(* Logix 5000 Program export KEP; software revision 30.00; part 11 of 15 *)
(* tags used below, declared in another part *)
   EdDSA_INTERNAL : EdDSA_INTERNAL[5];
   EdDSA_STATES : EdDSA_STATECTRL[15];
   InternalFlags : InternalFlags[5];
   InternalFlag_AllNodesUsingKsPrime : BOOL;
   InternalFlag_CreateNewKsPrime : BOOL;
   InternalFlag_KeyServerIdentityNo : BOOL;
   InternalFlag_KeyServerIdentityYes : BOOL;
   InternalFlag_KsEqualKsPrimeStatus : BOOL;
   InternalFlag_KsExists : BOOL;
   InternalFlag_KsIDMatchesServer : BOOL;
   InternalFlag_KsPrimeAvail : BOOL;
   InternalFlag_KsPrimeExists : BOOL;
   InternalFlag_KsPrimeIDMatchesServer : BOOL;
   InternalFlag_PowerOnCycle : BOOL;
   Internal_EdDSA_Msg : EdDSA_MSG;
   KsPrimeExchangeErrorTimer : TIMER;
   MyNodeNumber : DINT;
   ProcessorState : DINT;
   ServerNode : INT;
   T_INT1 : INT;
   WorkingNode : DINT;
   EdDSA_KS : DINT[8];
   EdDSA_KS_Prime : DINT[8];
   EdDSA_MSG_NODE_BLANK : EdDSA_MSG;
   EdDSA_MSG_TO_NODE1 : EdDSA_MSG;
   EdDSA_MSG_TO_NODE2 : EdDSA_MSG;
   EdDSA_MSG_TO_NODE3 : EdDSA_MSG;
   EdDSA_MSG_TO_NODE4 : EdDSA_MSG;
   FirstScan_EdDSA : BOOL;
   InternalFlag_AllNodesHaveMyKs : BOOL;
   InternalFlag_AllNodesHaveMyKsPrime : BOOL;
   InternalFlag_KsID : LINT;
   InternalFlag_KsPrimeID : LINT;
   NODE : VMAC_DATA_INTERNAL[5];
   Wrk_InpA : DINT[2];
   Wrk_InpB : DINT[2];
(* KEP, continued *)

ROUTINE MainRoutine   (* ladder *)
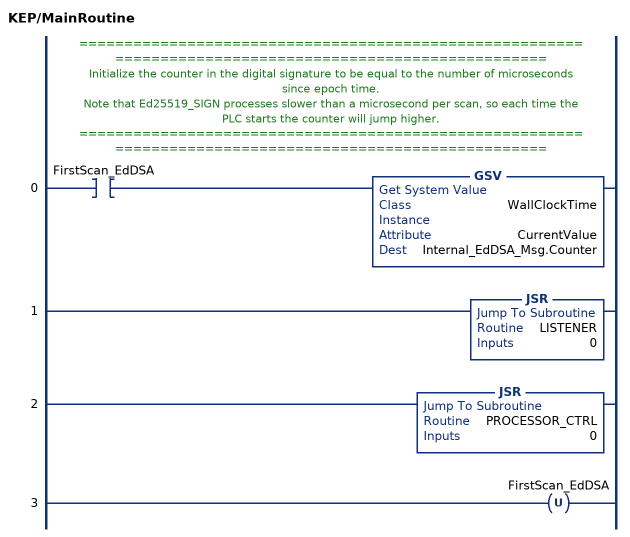
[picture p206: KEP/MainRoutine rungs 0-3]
   // ========================================================================================================
   // Initialize the counter in the digital signature to be equal to the number of microseconds since epoch time.
   // Note that Ed25519_SIGN processes slower than a microsecond per scan, so each time the PLC starts the counter will jump higher.
   // ========================================================================================================
   0: XIC(FirstScan_EdDSA)GSV(WallClockTime,,CurrentValue,Internal_EdDSA_Msg.Counter);
   1: JSR(LISTENER,0);
   2: JSR(PROCESSOR_CTRL,0);
   3: OTU(FirstScan_EdDSA);
END_ROUTINE

ROUTINE PROCESSOR_CTRL   (* ladder *)
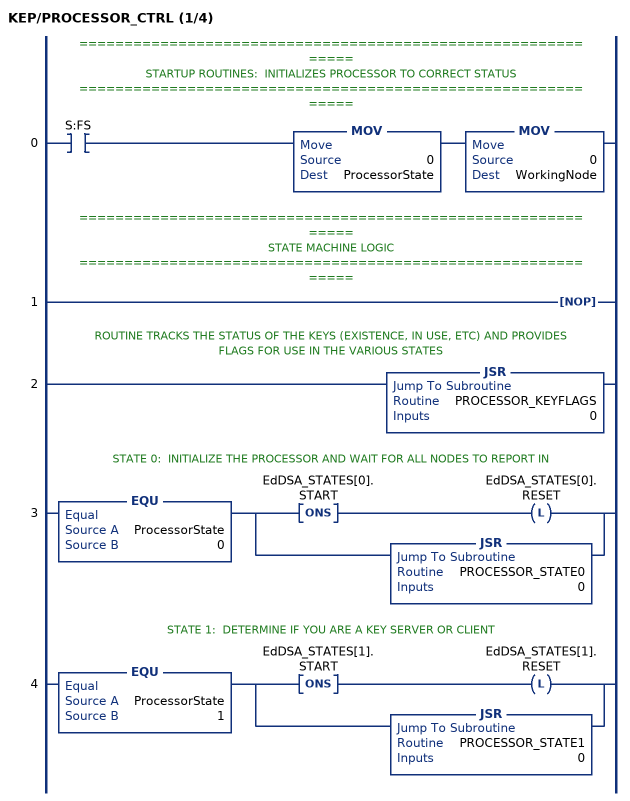
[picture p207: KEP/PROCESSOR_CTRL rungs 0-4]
   // =============================================================
   // STARTUP ROUTINES:  INITIALIZES PROCESSOR TO CORRECT STATUS
   // =============================================================
   0: XIC(S:FS)MOV(0,ProcessorState)MOV(0,WorkingNode);
   // =============================================================
   // STATE MACHINE LOGIC
   // =============================================================
   1: NOP();
   // ROUTINE TRACKS THE STATUS OF THE KEYS (EXISTENCE, IN USE, ETC) AND PROVIDES FLAGS FOR USE IN THE VARIOUS STATES
   2: JSR(PROCESSOR_KEYFLAGS,0);
   // STATE 0:  INITIALIZE THE PROCESSOR AND WAIT FOR ALL NODES TO REPORT IN
   3: EQU(ProcessorState,0)[ONS(EdDSA_STATES[0].START) OTL(EdDSA_STATES[0].RESET) ,JSR(PROCESSOR_STATE0,0) ];
   // STATE 1:  DETERMINE IF YOU ARE A KEY SERVER OR CLIENT
   4: EQU(ProcessorState,1)[ONS(EdDSA_STATES[1].START) OTL(EdDSA_STATES[1].RESET) ,JSR(PROCESSOR_STATE1,0) ];
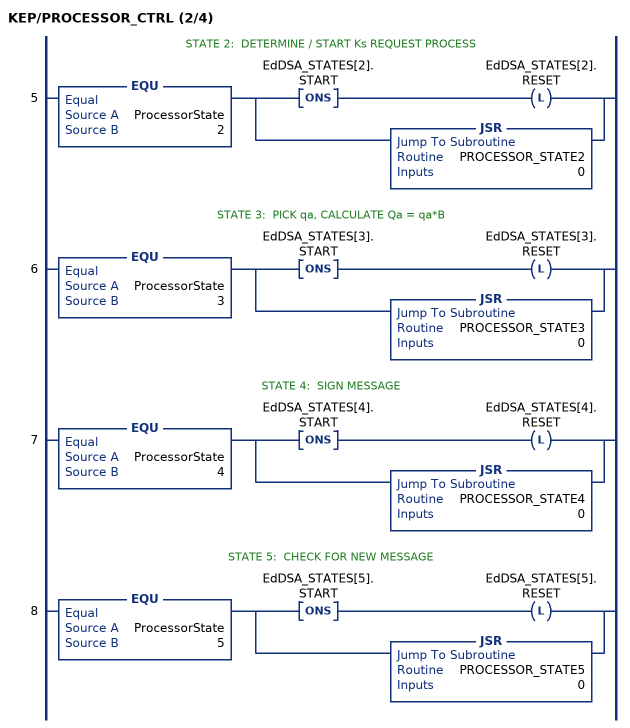
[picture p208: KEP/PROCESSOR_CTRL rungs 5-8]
   // STATE 2:  DETERMINE / START Ks REQUEST PROCESS
   5: EQU(ProcessorState,2)[ONS(EdDSA_STATES[2].START) OTL(EdDSA_STATES[2].RESET) ,JSR(PROCESSOR_STATE2,0) ];
   // STATE 3:  PICK qa, CALCULATE Qa = qa*B
   6: EQU(ProcessorState,3)[ONS(EdDSA_STATES[3].START) OTL(EdDSA_STATES[3].RESET) ,JSR(PROCESSOR_STATE3,0) ];
   // STATE 4:  SIGN MESSAGE
   7: EQU(ProcessorState,4)[ONS(EdDSA_STATES[4].START) OTL(EdDSA_STATES[4].RESET) ,JSR(PROCESSOR_STATE4,0) ];
   // STATE 5:  CHECK FOR NEW MESSAGE
   8: EQU(ProcessorState,5)[ONS(EdDSA_STATES[5].START) OTL(EdDSA_STATES[5].RESET) ,JSR(PROCESSOR_STATE5,0) ];
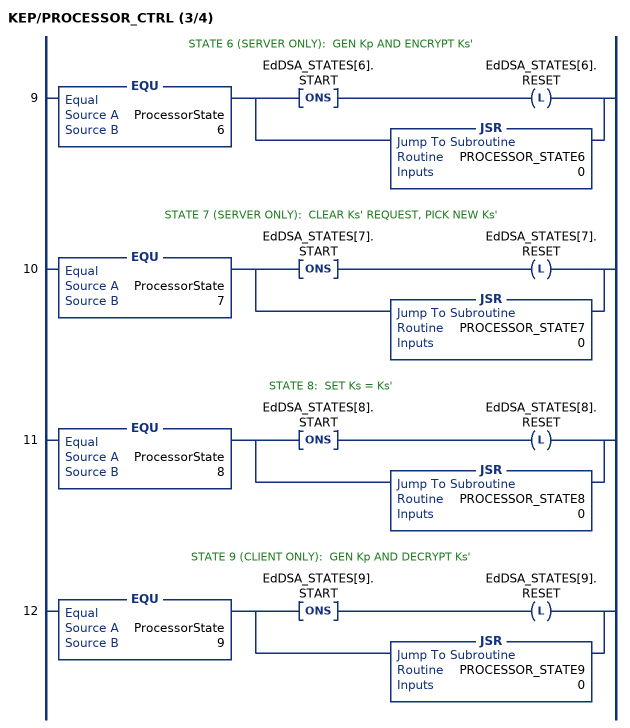
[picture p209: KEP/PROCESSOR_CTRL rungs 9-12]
   // STATE 6 (SERVER ONLY):  GEN Kp AND ENCRYPT Ks'
   9: EQU(ProcessorState,6)[ONS(EdDSA_STATES[6].START) OTL(EdDSA_STATES[6].RESET) ,JSR(PROCESSOR_STATE6,0) ];
   // STATE 7 (SERVER ONLY):  CLEAR Ks' REQUEST, PICK NEW Ks'
   10: EQU(ProcessorState,7)[ONS(EdDSA_STATES[7].START) OTL(EdDSA_STATES[7].RESET) ,JSR(PROCESSOR_STATE7,0) ];
   // STATE 8:  SET Ks = Ks'
   11: EQU(ProcessorState,8)[ONS(EdDSA_STATES[8].START) OTL(EdDSA_STATES[8].RESET) ,JSR(PROCESSOR_STATE8,0) ];
   // STATE 9 (CLIENT ONLY):  GEN Kp AND DECRYPT Ks'
   12: EQU(ProcessorState,9)[ONS(EdDSA_STATES[9].START) OTL(EdDSA_STATES[9].RESET) ,JSR(PROCESSOR_STATE9,0) ];
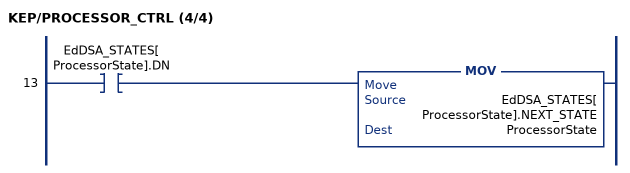
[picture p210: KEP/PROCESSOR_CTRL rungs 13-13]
   13: XIC(EdDSA_STATES[ProcessorState].DN)MOV(EdDSA_STATES[ProcessorState].NEXT_STATE,ProcessorState);
END_ROUTINE

ROUTINE PROCESSOR_KEYFLAGS   (* ladder *)
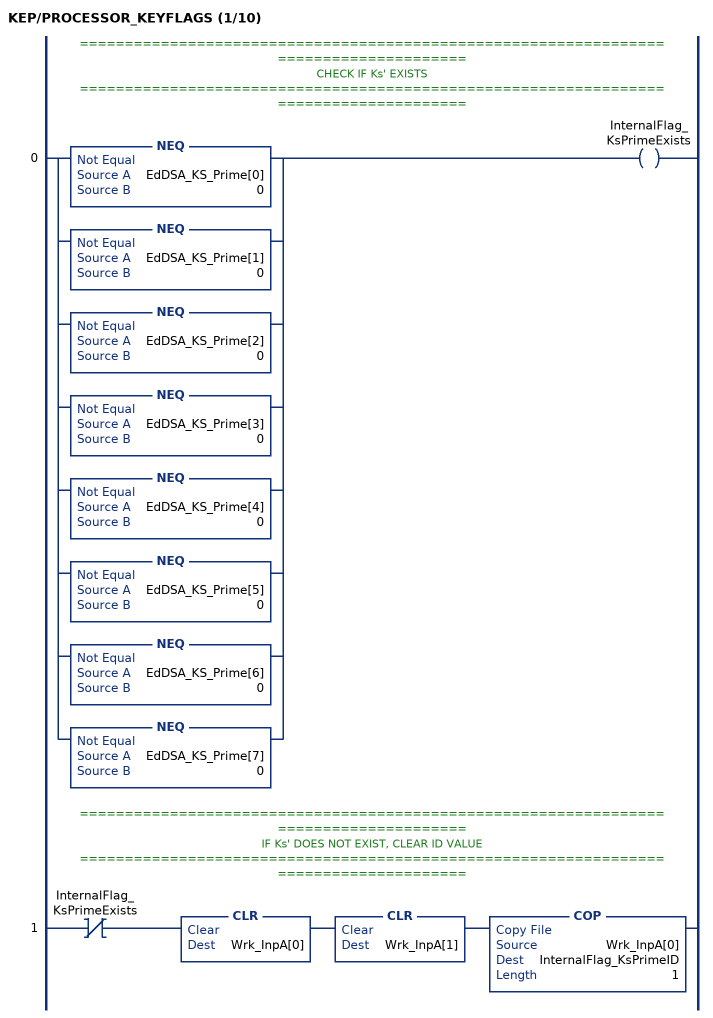
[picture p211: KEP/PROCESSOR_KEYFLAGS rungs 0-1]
   // ======================================================================================
   // CHECK IF Ks' EXISTS
   // ======================================================================================
   0: [NEQ(EdDSA_KS_Prime[0],0) ,NEQ(EdDSA_KS_Prime[1],0) ,NEQ(EdDSA_KS_Prime[2],0) ,NEQ(EdDSA_KS_Prime[3],0) ,NEQ(EdDSA_KS_Prime[4],0) ,NEQ(EdDSA_KS_Prime[5],0) ,NEQ(EdDSA_KS_Prime[6],0) ,NEQ(EdDSA_KS_Prime[7],0) ]OTE(InternalFlag_KsPrimeExists);
   // ======================================================================================
   // IF Ks' DOES NOT EXIST, CLEAR ID VALUE
   // ======================================================================================
   1: XIO(InternalFlag_KsPrimeExists)CLR(Wrk_InpA[0])CLR(Wrk_InpA[1])COP(Wrk_InpA[0],InternalFlag_KsPrimeID,1);
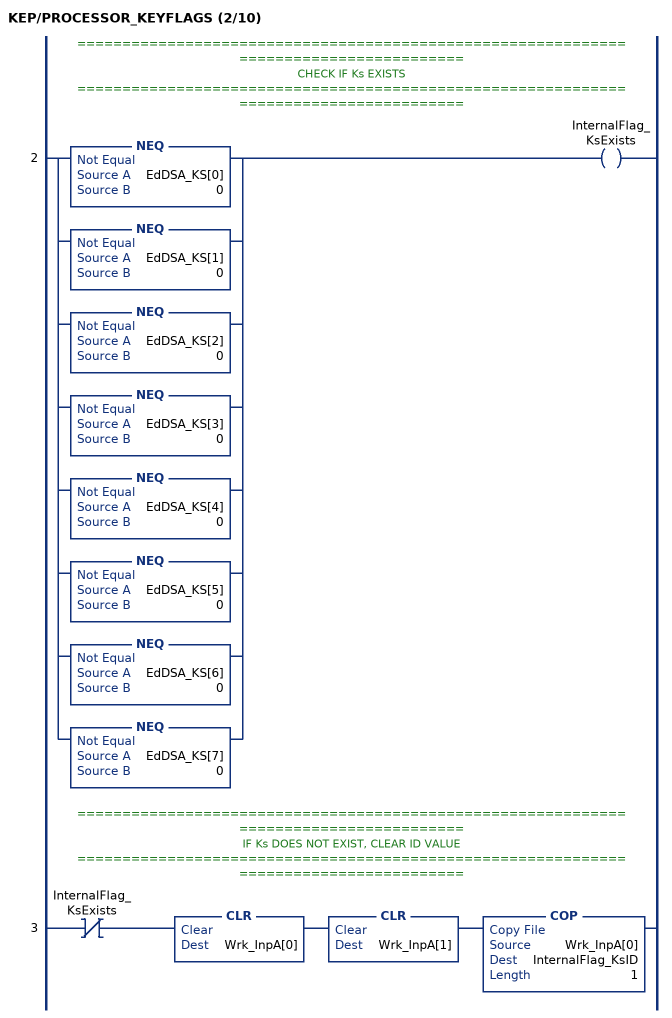
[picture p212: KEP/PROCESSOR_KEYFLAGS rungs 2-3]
   // ======================================================================================
   // CHECK IF Ks EXISTS
   // ======================================================================================
   2: [NEQ(EdDSA_KS[0],0) ,NEQ(EdDSA_KS[1],0) ,NEQ(EdDSA_KS[2],0) ,NEQ(EdDSA_KS[3],0) ,NEQ(EdDSA_KS[4],0) ,NEQ(EdDSA_KS[5],0) ,NEQ(EdDSA_KS[6],0) ,NEQ(EdDSA_KS[7],0) ]OTE(InternalFlag_KsExists);
   // ======================================================================================
   // IF Ks DOES NOT EXIST, CLEAR ID VALUE
   // ======================================================================================
   3: XIO(InternalFlag_KsExists)CLR(Wrk_InpA[0])CLR(Wrk_InpA[1])COP(Wrk_InpA[0],InternalFlag_KsID,1);
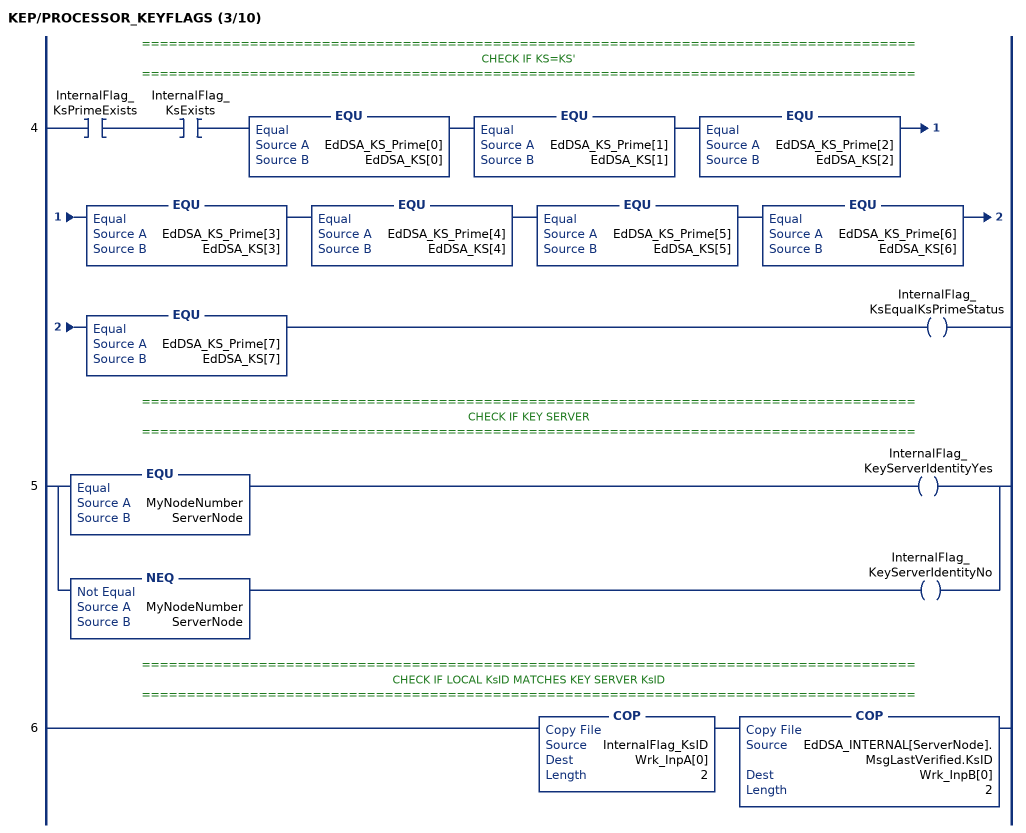
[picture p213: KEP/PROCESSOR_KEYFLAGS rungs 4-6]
   // ======================================================================================
   // CHECK IF KS=KS'
   // ======================================================================================
   4: XIC(InternalFlag_KsPrimeExists)XIC(InternalFlag_KsExists)EQU(EdDSA_KS_Prime[0],EdDSA_KS[0])EQU(EdDSA_KS_Prime[1],EdDSA_KS[1])EQU(EdDSA_KS_Prime[2],EdDSA_KS[2])EQU(EdDSA_KS_Prime[3],EdDSA_KS[3])EQU(EdDSA_KS_Prime[4],EdDSA_KS[4])EQU(EdDSA_KS_Prime[5],EdDSA_KS[5])EQU(EdDSA_KS_Prime[6],EdDSA_KS[6])EQU(EdDSA_KS_Prime[7],EdDSA_KS[7])OTE(InternalFlag_KsEqualKsPrimeStatus);
   // ======================================================================================
   // CHECK IF KEY SERVER
   // ======================================================================================
   5: [EQU(MyNodeNumber,ServerNode) OTE(InternalFlag_KeyServerIdentityYes) ,NEQ(MyNodeNumber,ServerNode) OTE(InternalFlag_KeyServerIdentityNo) ];
   // ======================================================================================
   // CHECK IF LOCAL KsID MATCHES KEY SERVER KsID
   // ======================================================================================
   6: COP(InternalFlag_KsID,Wrk_InpA[0],2)COP(EdDSA_INTERNAL[ServerNode].MsgLastVerified.KsID,Wrk_InpB[0],2);
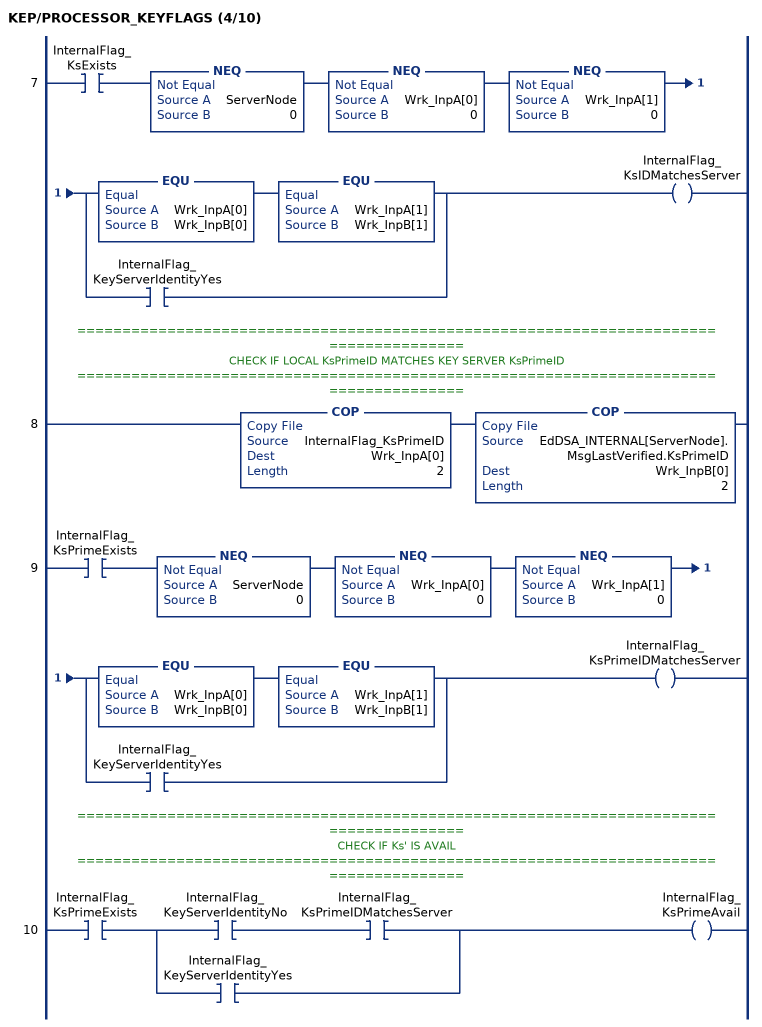
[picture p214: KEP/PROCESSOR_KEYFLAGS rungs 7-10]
   7: XIC(InternalFlag_KsExists)NEQ(ServerNode,0)NEQ(Wrk_InpA[0],0)NEQ(Wrk_InpA[1],0)[EQU(Wrk_InpA[0],Wrk_InpB[0]) EQU(Wrk_InpA[1],Wrk_InpB[1]) ,XIC(InternalFlag_KeyServerIdentityYes) ]OTE(InternalFlag_KsIDMatchesServer);
   // ======================================================================================
   // CHECK IF LOCAL KsPrimeID MATCHES KEY SERVER KsPrimeID
   // ======================================================================================
   8: COP(InternalFlag_KsPrimeID,Wrk_InpA[0],2)COP(EdDSA_INTERNAL[ServerNode].MsgLastVerified.KsPrimeID,Wrk_InpB[0],2);
   9: XIC(InternalFlag_KsPrimeExists)NEQ(ServerNode,0)NEQ(Wrk_InpA[0],0)NEQ(Wrk_InpA[1],0)[EQU(Wrk_InpA[0],Wrk_InpB[0]) EQU(Wrk_InpA[1],Wrk_InpB[1]) ,XIC(InternalFlag_KeyServerIdentityYes) ]OTE(InternalFlag_KsPrimeIDMatchesServer);
   // ======================================================================================
   // CHECK IF Ks' IS AVAIL
   // ======================================================================================
   10: XIC(InternalFlag_KsPrimeExists)[XIC(InternalFlag_KeyServerIdentityNo) XIC(InternalFlag_KsPrimeIDMatchesServer) ,XIC(InternalFlag_KeyServerIdentityYes) ]OTE(InternalFlag_KsPrimeAvail);
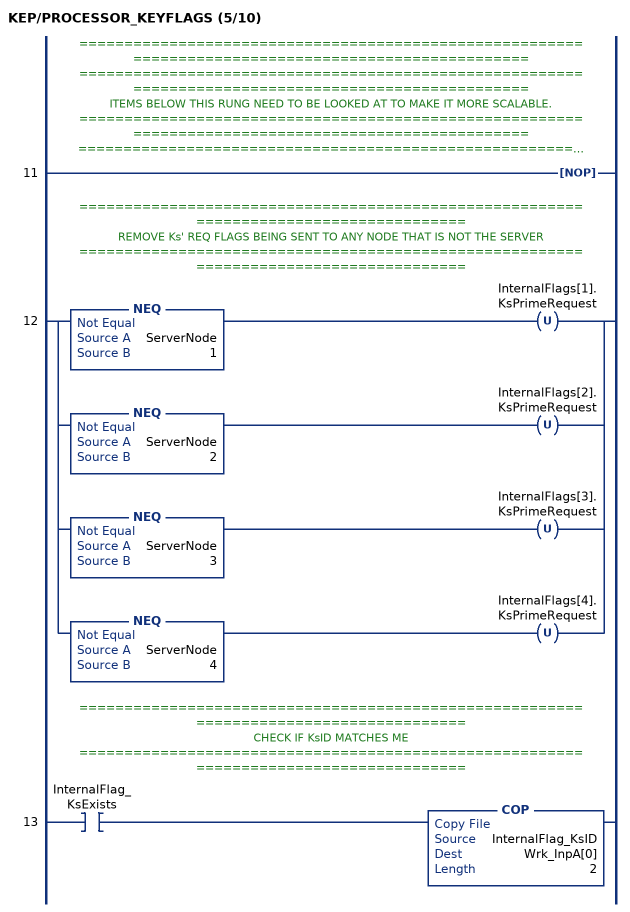
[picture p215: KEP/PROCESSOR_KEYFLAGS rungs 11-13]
   // ====================================================================================================
   // ====================================================================================================
   // ITEMS BELOW THIS RUNG NEED TO BE LOOKED AT TO MAKE IT MORE SCALABLE.
   // ====================================================================================================
   // ====================================================================================================
   11: NOP();
   // ======================================================================================
   // REMOVE Ks' REQ FLAGS BEING SENT TO ANY NODE THAT IS NOT THE SERVER
   // ======================================================================================
   12: [NEQ(ServerNode,1) OTU(InternalFlags[1].KsPrimeRequest) ,NEQ(ServerNode,2) OTU(InternalFlags[2].KsPrimeRequest) ,NEQ(ServerNode,3) OTU(InternalFlags[3].KsPrimeRequest) ,NEQ(ServerNode,4) OTU(InternalFlags[4].KsPrimeRequest) ];
   // ======================================================================================
   // CHECK IF KsID MATCHES ME
   // ======================================================================================
   13: XIC(InternalFlag_KsExists)COP(InternalFlag_KsID,Wrk_InpA[0],2);
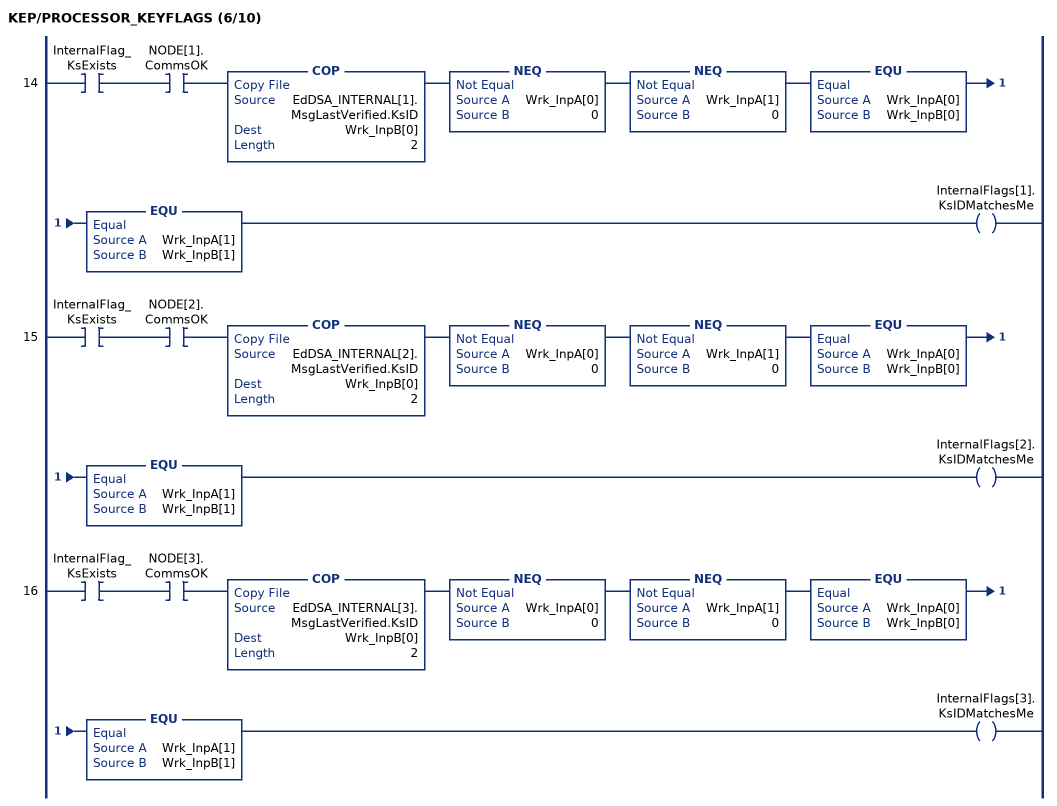
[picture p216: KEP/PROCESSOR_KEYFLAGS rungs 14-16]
   14: XIC(InternalFlag_KsExists)XIC(NODE[1].CommsOK)COP(EdDSA_INTERNAL[1].MsgLastVerified.KsID,Wrk_InpB[0],2)NEQ(Wrk_InpA[0],0)NEQ(Wrk_InpA[1],0)EQU(Wrk_InpA[0],Wrk_InpB[0])EQU(Wrk_InpA[1],Wrk_InpB[1])OTE(InternalFlags[1].KsIDMatchesMe);
   15: XIC(InternalFlag_KsExists)XIC(NODE[2].CommsOK)COP(EdDSA_INTERNAL[2].MsgLastVerified.KsID,Wrk_InpB[0],2)NEQ(Wrk_InpA[0],0)NEQ(Wrk_InpA[1],0)EQU(Wrk_InpA[0],Wrk_InpB[0])EQU(Wrk_InpA[1],Wrk_InpB[1])OTE(InternalFlags[2].KsIDMatchesMe);
   16: XIC(InternalFlag_KsExists)XIC(NODE[3].CommsOK)COP(EdDSA_INTERNAL[3].MsgLastVerified.KsID,Wrk_InpB[0],2)NEQ(Wrk_InpA[0],0)NEQ(Wrk_InpA[1],0)EQU(Wrk_InpA[0],Wrk_InpB[0])EQU(Wrk_InpA[1],Wrk_InpB[1])OTE(InternalFlags[3].KsIDMatchesMe);
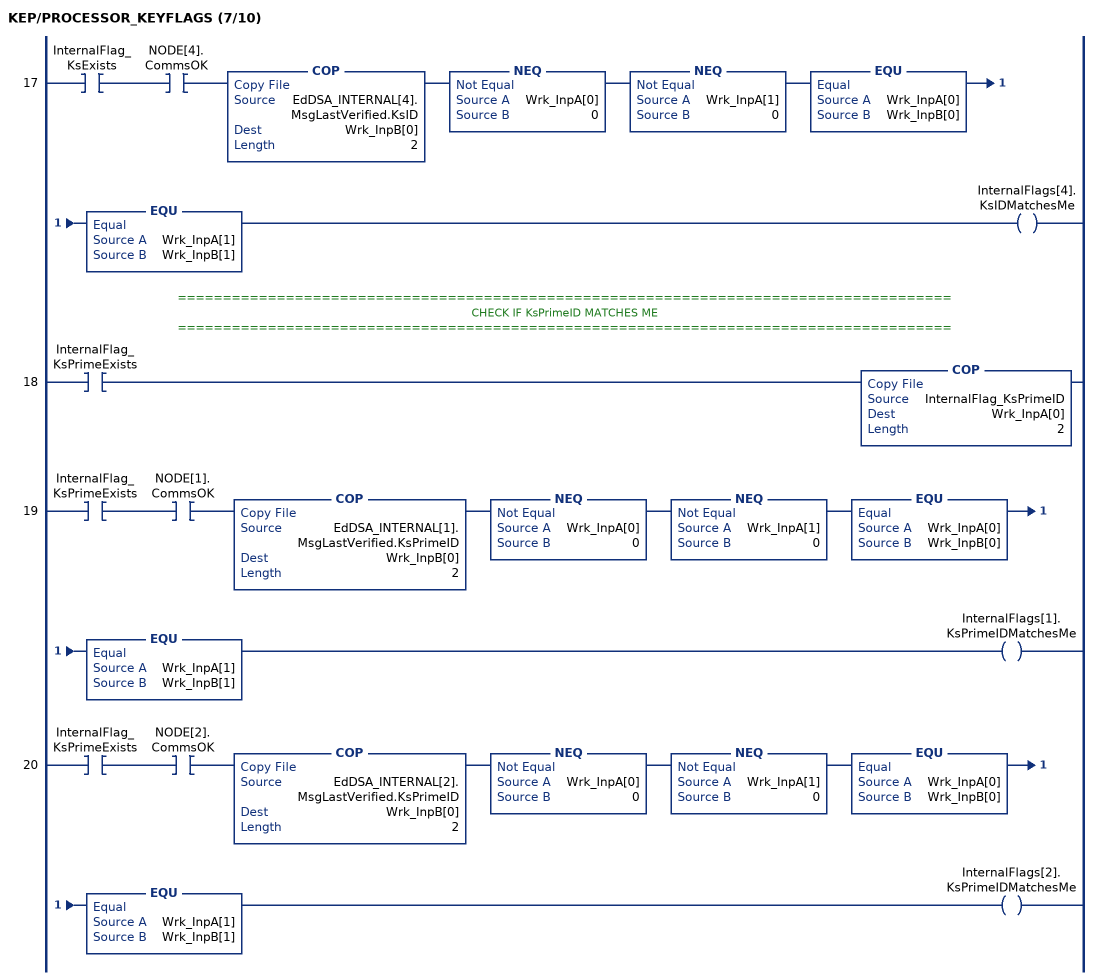
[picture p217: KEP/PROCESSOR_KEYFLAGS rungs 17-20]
   17: XIC(InternalFlag_KsExists)XIC(NODE[4].CommsOK)COP(EdDSA_INTERNAL[4].MsgLastVerified.KsID,Wrk_InpB[0],2)NEQ(Wrk_InpA[0],0)NEQ(Wrk_InpA[1],0)EQU(Wrk_InpA[0],Wrk_InpB[0])EQU(Wrk_InpA[1],Wrk_InpB[1])OTE(InternalFlags[4].KsIDMatchesMe);
   // ======================================================================================
   // CHECK IF KsPrimeID MATCHES ME
   // ======================================================================================
   18: XIC(InternalFlag_KsPrimeExists)COP(InternalFlag_KsPrimeID,Wrk_InpA[0],2);
   19: XIC(InternalFlag_KsPrimeExists)XIC(NODE[1].CommsOK)COP(EdDSA_INTERNAL[1].MsgLastVerified.KsPrimeID,Wrk_InpB[0],2)NEQ(Wrk_InpA[0],0)NEQ(Wrk_InpA[1],0)EQU(Wrk_InpA[0],Wrk_InpB[0])EQU(Wrk_InpA[1],Wrk_InpB[1])OTE(InternalFlags[1].KsPrimeIDMatchesMe);
   20: XIC(InternalFlag_KsPrimeExists)XIC(NODE[2].CommsOK)COP(EdDSA_INTERNAL[2].MsgLastVerified.KsPrimeID,Wrk_InpB[0],2)NEQ(Wrk_InpA[0],0)NEQ(Wrk_InpA[1],0)EQU(Wrk_InpA[0],Wrk_InpB[0])EQU(Wrk_InpA[1],Wrk_InpB[1])OTE(InternalFlags[2].KsPrimeIDMatchesMe);
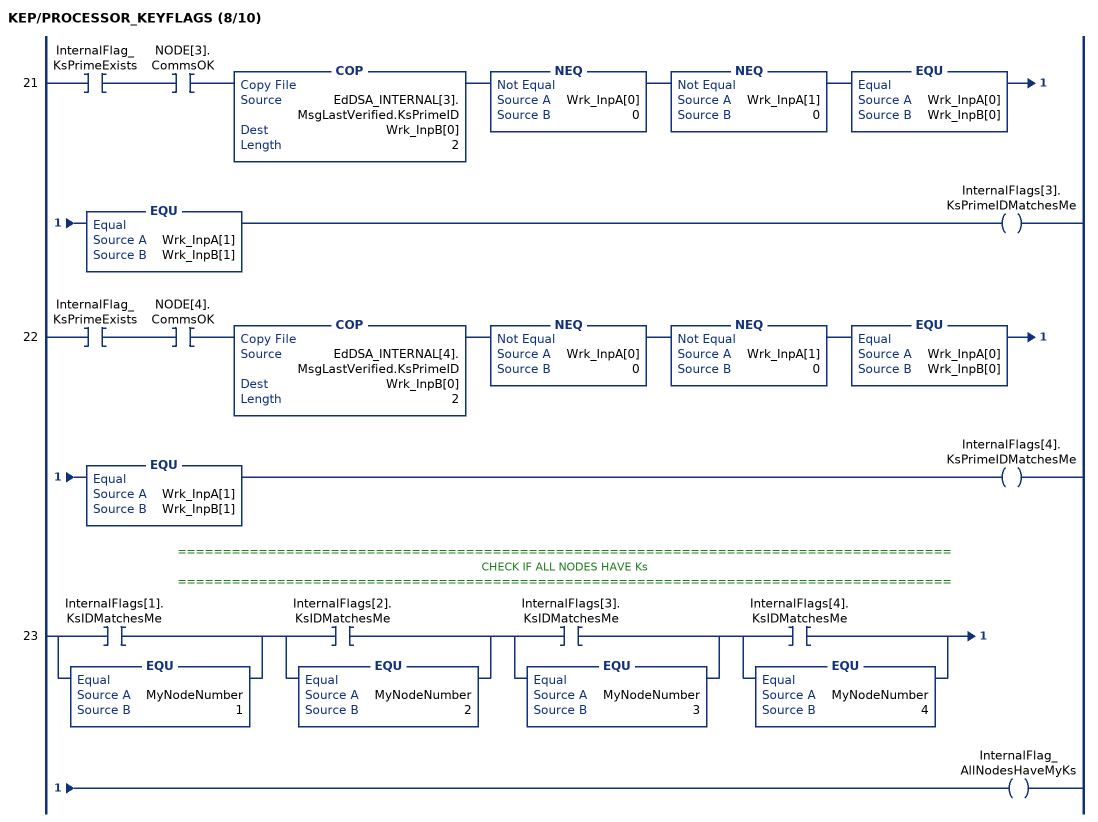
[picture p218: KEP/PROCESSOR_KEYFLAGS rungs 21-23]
   21: XIC(InternalFlag_KsPrimeExists)XIC(NODE[3].CommsOK)COP(EdDSA_INTERNAL[3].MsgLastVerified.KsPrimeID,Wrk_InpB[0],2)NEQ(Wrk_InpA[0],0)NEQ(Wrk_InpA[1],0)EQU(Wrk_InpA[0],Wrk_InpB[0])EQU(Wrk_InpA[1],Wrk_InpB[1])OTE(InternalFlags[3].KsPrimeIDMatchesMe);
   22: XIC(InternalFlag_KsPrimeExists)XIC(NODE[4].CommsOK)COP(EdDSA_INTERNAL[4].MsgLastVerified.KsPrimeID,Wrk_InpB[0],2)NEQ(Wrk_InpA[0],0)NEQ(Wrk_InpA[1],0)EQU(Wrk_InpA[0],Wrk_InpB[0])EQU(Wrk_InpA[1],Wrk_InpB[1])OTE(InternalFlags[4].KsPrimeIDMatchesMe);
   // ======================================================================================
   // CHECK IF ALL NODES HAVE Ks
   // ======================================================================================
   23: [XIC(InternalFlags[1].KsIDMatchesMe) ,EQU(MyNodeNumber,1) ][XIC(InternalFlags[2].KsIDMatchesMe) ,EQU(MyNodeNumber,2) ][XIC(InternalFlags[3].KsIDMatchesMe) ,EQU(MyNodeNumber,3) ][XIC(InternalFlags[4].KsIDMatchesMe) ,EQU(MyNodeNumber,4) ]OTE(InternalFlag_AllNodesHaveMyKs);
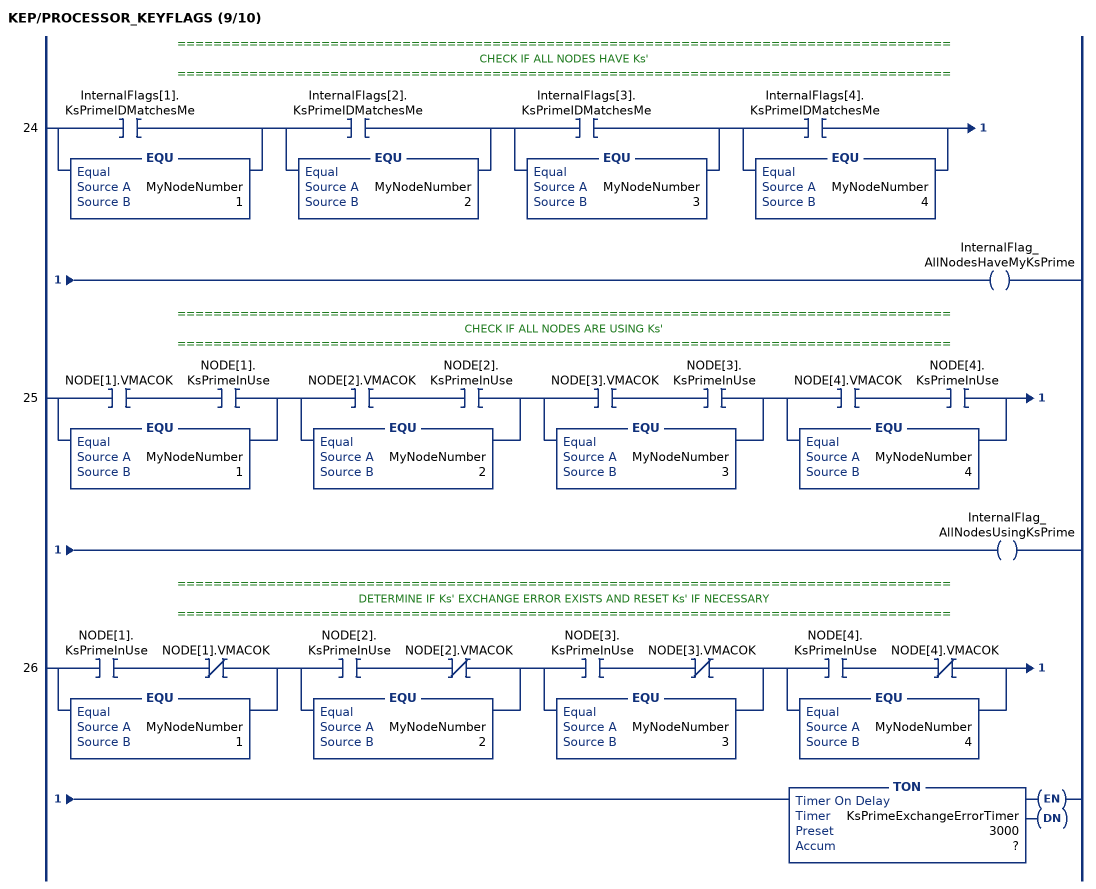
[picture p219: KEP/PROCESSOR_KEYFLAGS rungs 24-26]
   // ======================================================================================
   // CHECK IF ALL NODES HAVE Ks'
   // ======================================================================================
   24: [XIC(InternalFlags[1].KsPrimeIDMatchesMe) ,EQU(MyNodeNumber,1) ][XIC(InternalFlags[2].KsPrimeIDMatchesMe) ,EQU(MyNodeNumber,2) ][XIC(InternalFlags[3].KsPrimeIDMatchesMe) ,EQU(MyNodeNumber,3) ][XIC(InternalFlags[4].KsPrimeIDMatchesMe) ,EQU(MyNodeNumber,4) ]OTE(InternalFlag_AllNodesHaveMyKsPrime);
   // ======================================================================================
   // CHECK IF ALL NODES ARE USING Ks'
   // ======================================================================================
   25: [XIC(NODE[1].VMACOK) XIC(NODE[1].KsPrimeInUse) ,EQU(MyNodeNumber,1) ][XIC(NODE[2].VMACOK) XIC(NODE[2].KsPrimeInUse) ,EQU(MyNodeNumber,2) ][XIC(NODE[3].VMACOK) XIC(NODE[3].KsPrimeInUse) ,EQU(MyNodeNumber,3) ][XIC(NODE[4].VMACOK) XIC(NODE[4].KsPrimeInUse) ,EQU(MyNodeNumber,4) ]OTE(InternalFlag_AllNodesUsingKsPrime);
   // ======================================================================================
   // DETERMINE IF Ks' EXCHANGE ERROR EXISTS AND RESET Ks' IF NECESSARY
   // ======================================================================================
   26: [XIC(NODE[1].KsPrimeInUse) XIO(NODE[1].VMACOK) ,EQU(MyNodeNumber,1) ][XIC(NODE[2].KsPrimeInUse) XIO(NODE[2].VMACOK) ,EQU(MyNodeNumber,2) ][XIC(NODE[3].KsPrimeInUse) XIO(NODE[3].VMACOK) ,EQU(MyNodeNumber,3) ][XIC(NODE[4].KsPrimeInUse) XIO(NODE[4].VMACOK) ,EQU(MyNodeNumber,4) ]TON(KsPrimeExchangeErrorTimer,?,?);
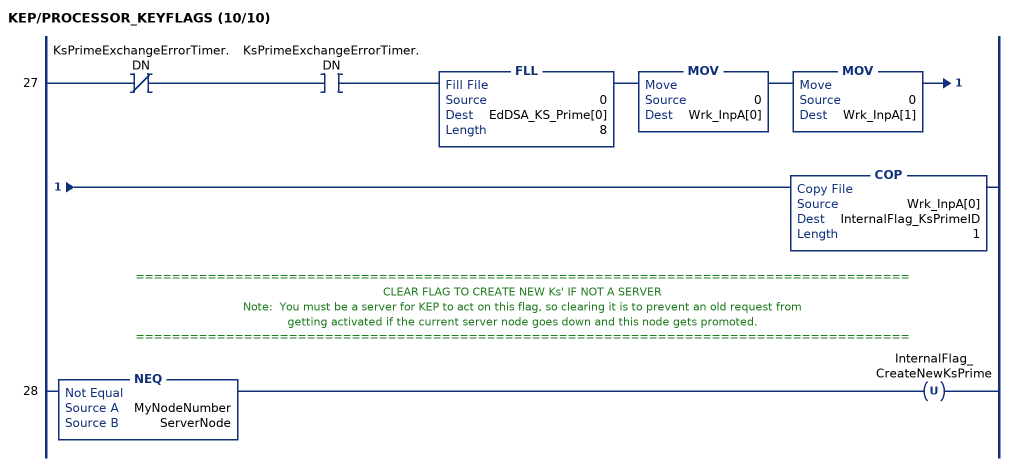
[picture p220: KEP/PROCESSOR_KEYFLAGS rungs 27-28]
   27: XIO(KsPrimeExchangeErrorTimer.DN)XIC(KsPrimeExchangeErrorTimer.DN)FLL(0,EdDSA_KS_Prime[0],8)MOV(0,Wrk_InpA[0])MOV(0,Wrk_InpA[1])COP(Wrk_InpA[0],InternalFlag_KsPrimeID,1);
   // ======================================================================================
   // CLEAR FLAG TO CREATE NEW Ks' IF NOT A SERVER
   // Note:  You must be a server for KEP to act on this flag, so clearing it is to prevent an old request from
   // getting activated if the current server node goes down and this node gets promoted.
   // ======================================================================================
   28: NEQ(MyNodeNumber,ServerNode)OTU(InternalFlag_CreateNewKsPrime);
END_ROUTINE

ROUTINE PROCESSOR_STATE0   (* ladder *)
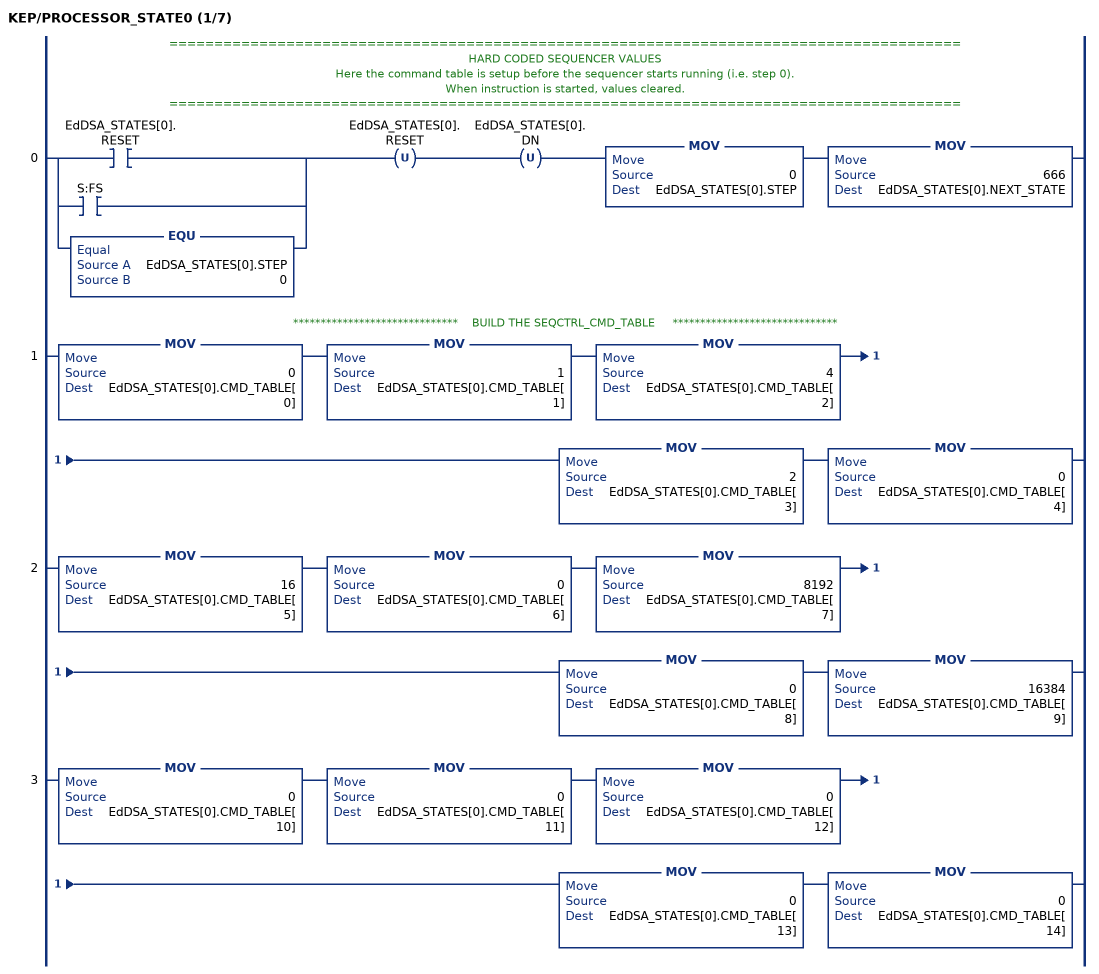
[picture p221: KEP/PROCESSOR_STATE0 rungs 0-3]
   // ========================================================================================
   // HARD CODED SEQUENCER VALUES
   // Here the command table is setup before the sequencer starts running (i.e. step 0).
   // When instruction is started, values cleared.
   // ========================================================================================
   0: [[XIC(EdDSA_STATES[0].RESET) ,XIC(S:FS) ] ,EQU(EdDSA_STATES[0].STEP,0) ]OTU(EdDSA_STATES[0].RESET)OTU(EdDSA_STATES[0].DN)MOV(0,EdDSA_STATES[0].STEP)MOV(666,EdDSA_STATES[0].NEXT_STATE);
   // ******************************    BUILD THE SEQCTRL_CMD_TABLE     ******************************
   1: MOV(0,EdDSA_STATES[0].CMD_TABLE[0])MOV(1,EdDSA_STATES[0].CMD_TABLE[1])MOV(4,EdDSA_STATES[0].CMD_TABLE[2])MOV(2,EdDSA_STATES[0].CMD_TABLE[3])MOV(0,EdDSA_STATES[0].CMD_TABLE[4]);
   2: MOV(16,EdDSA_STATES[0].CMD_TABLE[5])MOV(0,EdDSA_STATES[0].CMD_TABLE[6])MOV(8192,EdDSA_STATES[0].CMD_TABLE[7])MOV(0,EdDSA_STATES[0].CMD_TABLE[8])MOV(16384,EdDSA_STATES[0].CMD_TABLE[9]);
   3: MOV(0,EdDSA_STATES[0].CMD_TABLE[10])MOV(0,EdDSA_STATES[0].CMD_TABLE[11])MOV(0,EdDSA_STATES[0].CMD_TABLE[12])MOV(0,EdDSA_STATES[0].CMD_TABLE[13])MOV(0,EdDSA_STATES[0].CMD_TABLE[14]);
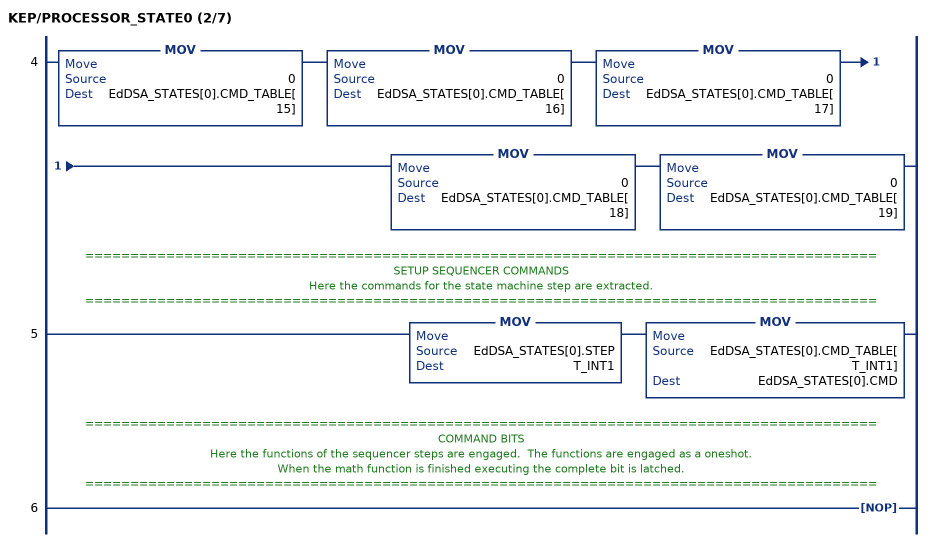
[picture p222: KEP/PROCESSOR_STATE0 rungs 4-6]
   4: MOV(0,EdDSA_STATES[0].CMD_TABLE[15])MOV(0,EdDSA_STATES[0].CMD_TABLE[16])MOV(0,EdDSA_STATES[0].CMD_TABLE[17])MOV(0,EdDSA_STATES[0].CMD_TABLE[18])MOV(0,EdDSA_STATES[0].CMD_TABLE[19]);
   // ========================================================================================
   // SETUP SEQUENCER COMMANDS
   // Here the commands for the state machine step are extracted.
   // ========================================================================================
   5: MOV(EdDSA_STATES[0].STEP,T_INT1)MOV(EdDSA_STATES[0].CMD_TABLE[T_INT1],EdDSA_STATES[0].CMD);
   // ========================================================================================
   // COMMAND BITS
   // Here the functions of the sequencer steps are engaged.  The functions are engaged as a oneshot.
   // When the math function is finished executing the complete bit is latched.
   // ========================================================================================
   6: NOP();
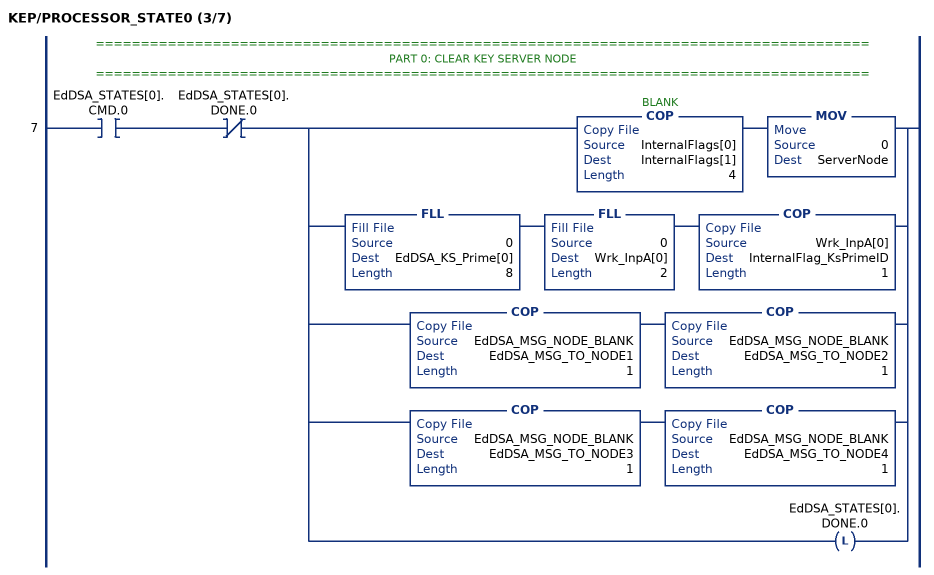
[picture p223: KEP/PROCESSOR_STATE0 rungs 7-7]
   // ======================================================================================
   // PART 0: CLEAR KEY SERVER NODE
   // ======================================================================================
   7: XIC(EdDSA_STATES[0].CMD.0)XIO(EdDSA_STATES[0].DONE.0)[COP(InternalFlags[0],InternalFlags[1],4) MOV(0,ServerNode) ,FLL(0,EdDSA_KS_Prime[0],8) FLL(0,Wrk_InpA[0],2) COP(Wrk_InpA[0],InternalFlag_KsPrimeID,1) ,COP(EdDSA_MSG_NODE_BLANK,EdDSA_MSG_TO_NODE1,1) COP(EdDSA_MSG_NODE_BLANK,EdDSA_MSG_TO_NODE2,1) ,COP(EdDSA_MSG_NODE_BLANK,EdDSA_MSG_TO_NODE3,1) COP(EdDSA_MSG_NODE_BLANK,EdDSA_MSG_TO_NODE4,1) ,OTL(EdDSA_STATES[0].DONE.0) ];
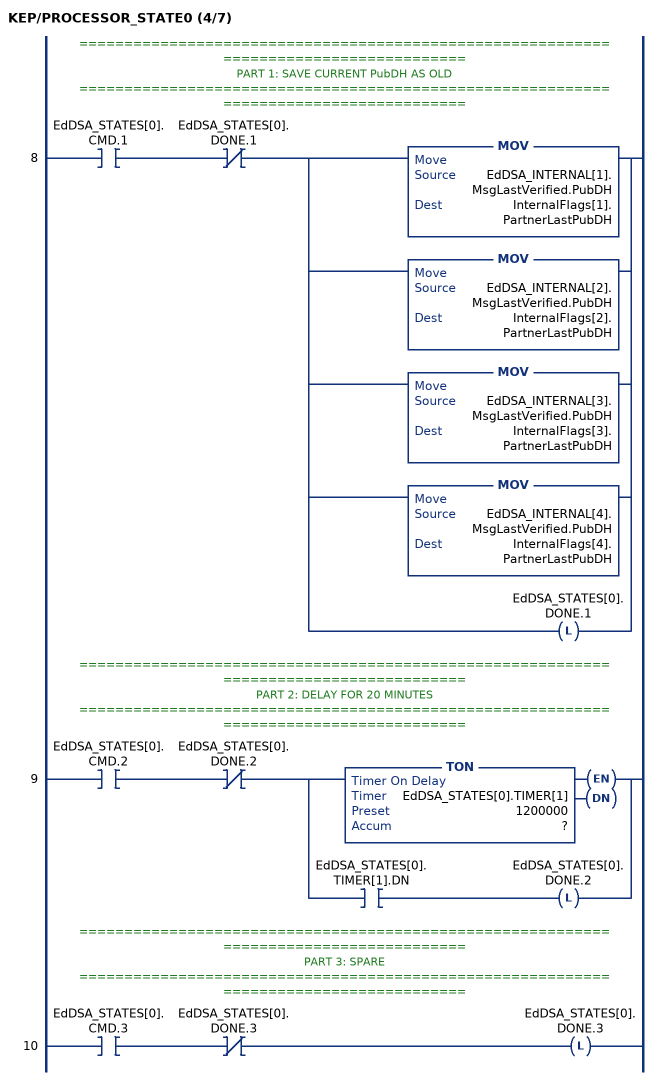
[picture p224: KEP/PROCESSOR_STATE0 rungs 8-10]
   // ======================================================================================
   // PART 1: SAVE CURRENT PubDH AS OLD
   // ======================================================================================
   8: XIC(EdDSA_STATES[0].CMD.1)XIO(EdDSA_STATES[0].DONE.1)[MOV(EdDSA_INTERNAL[1].MsgLastVerified.PubDH,InternalFlags[1].PartnerLastPubDH) ,MOV(EdDSA_INTERNAL[2].MsgLastVerified.PubDH,InternalFlags[2].PartnerLastPubDH) ,MOV(EdDSA_INTERNAL[3].MsgLastVerified.PubDH,InternalFlags[3].PartnerLastPubDH) ,MOV(EdDSA_INTERNAL[4].MsgLastVerified.PubDH,InternalFlags[4].PartnerLastPubDH) ,OTL(EdDSA_STATES[0].DONE.1) ];
   // ======================================================================================
   // PART 2: DELAY FOR 20 MINUTES
   // ======================================================================================
   9: XIC(EdDSA_STATES[0].CMD.2)XIO(EdDSA_STATES[0].DONE.2)[TON(EdDSA_STATES[0].TIMER[1],?,?) ,XIC(EdDSA_STATES[0].TIMER[1].DN) OTL(EdDSA_STATES[0].DONE.2) ];
   // ======================================================================================
   // PART 3: SPARE
   // ======================================================================================
   10: XIC(EdDSA_STATES[0].CMD.3)XIO(EdDSA_STATES[0].DONE.3)OTL(EdDSA_STATES[0].DONE.3);
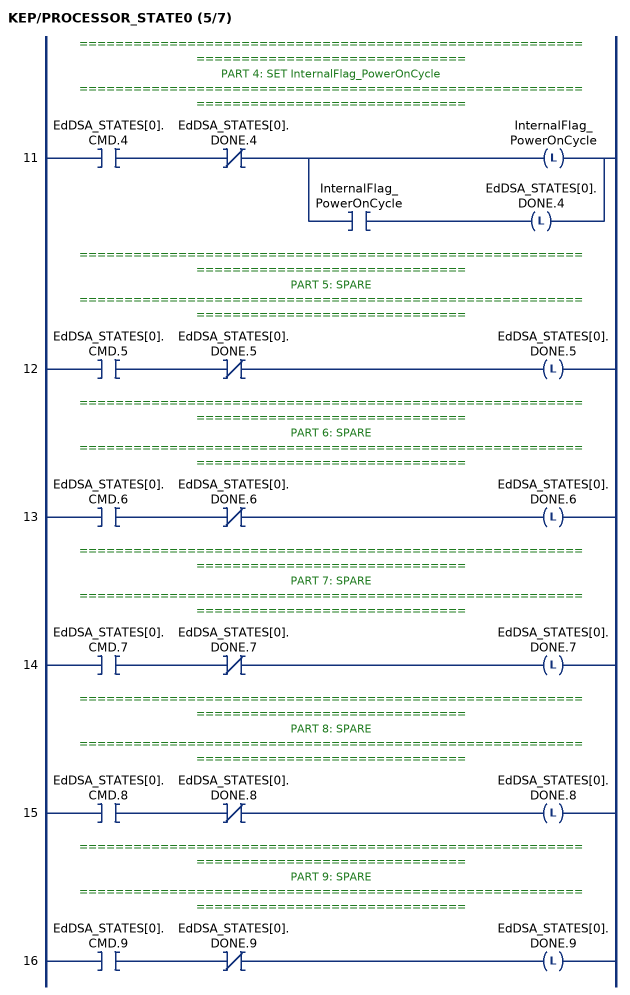
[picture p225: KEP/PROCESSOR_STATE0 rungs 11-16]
   // ======================================================================================
   // PART 4: SET InternalFlag_PowerOnCycle
   // ======================================================================================
   11: XIC(EdDSA_STATES[0].CMD.4)XIO(EdDSA_STATES[0].DONE.4)[OTL(InternalFlag_PowerOnCycle) ,XIC(InternalFlag_PowerOnCycle) OTL(EdDSA_STATES[0].DONE.4) ];
   // ======================================================================================
   // PART 5: SPARE
   // ======================================================================================
   12: XIC(EdDSA_STATES[0].CMD.5)XIO(EdDSA_STATES[0].DONE.5)OTL(EdDSA_STATES[0].DONE.5);
   // ======================================================================================
   // PART 6: SPARE
   // ======================================================================================
   13: XIC(EdDSA_STATES[0].CMD.6)XIO(EdDSA_STATES[0].DONE.6)OTL(EdDSA_STATES[0].DONE.6);
   // ======================================================================================
   // PART 7: SPARE
   // ======================================================================================
   14: XIC(EdDSA_STATES[0].CMD.7)XIO(EdDSA_STATES[0].DONE.7)OTL(EdDSA_STATES[0].DONE.7);
   // ======================================================================================
   // PART 8: SPARE
   // ======================================================================================
   15: XIC(EdDSA_STATES[0].CMD.8)XIO(EdDSA_STATES[0].DONE.8)OTL(EdDSA_STATES[0].DONE.8);
   // ======================================================================================
   // PART 9: SPARE
   // ======================================================================================
   16: XIC(EdDSA_STATES[0].CMD.9)XIO(EdDSA_STATES[0].DONE.9)OTL(EdDSA_STATES[0].DONE.9);
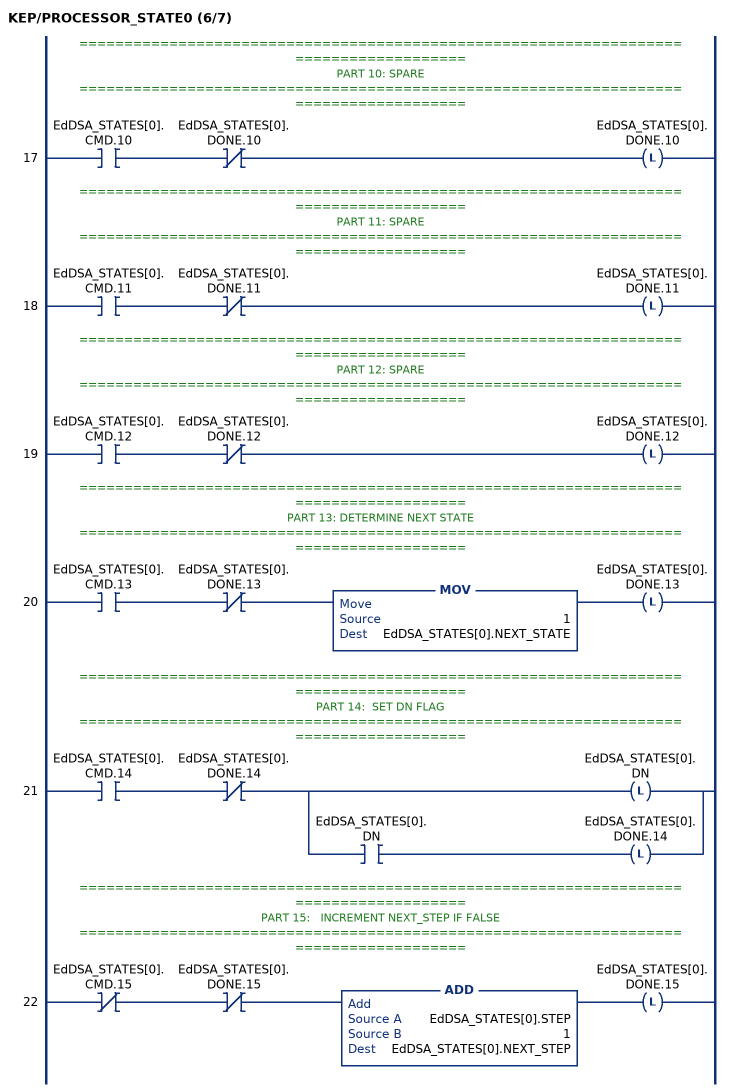
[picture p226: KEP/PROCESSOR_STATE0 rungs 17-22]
   // ======================================================================================
   // PART 10: SPARE
   // ======================================================================================
   17: XIC(EdDSA_STATES[0].CMD.10)XIO(EdDSA_STATES[0].DONE.10)OTL(EdDSA_STATES[0].DONE.10);
   // ======================================================================================
   // PART 11: SPARE
   // ======================================================================================
   18: XIC(EdDSA_STATES[0].CMD.11)XIO(EdDSA_STATES[0].DONE.11)OTL(EdDSA_STATES[0].DONE.11);
   // ======================================================================================
   // PART 12: SPARE
   // ======================================================================================
   19: XIC(EdDSA_STATES[0].CMD.12)XIO(EdDSA_STATES[0].DONE.12)OTL(EdDSA_STATES[0].DONE.12);
   // ======================================================================================
   // PART 13: DETERMINE NEXT STATE
   // ======================================================================================
   20: XIC(EdDSA_STATES[0].CMD.13)XIO(EdDSA_STATES[0].DONE.13)MOV(1,EdDSA_STATES[0].NEXT_STATE)OTL(EdDSA_STATES[0].DONE.13);
   // ======================================================================================
   // PART 14:  SET DN FLAG
   // ======================================================================================
   21: XIC(EdDSA_STATES[0].CMD.14)XIO(EdDSA_STATES[0].DONE.14)[OTL(EdDSA_STATES[0].DN) ,XIC(EdDSA_STATES[0].DN) OTL(EdDSA_STATES[0].DONE.14) ];
   // ======================================================================================
   // PART 15:   INCREMENT NEXT_STEP IF FALSE
   // ======================================================================================
   22: XIO(EdDSA_STATES[0].CMD.15)XIO(EdDSA_STATES[0].DONE.15)ADD(EdDSA_STATES[0].STEP,1,EdDSA_STATES[0].NEXT_STEP)OTL(EdDSA_STATES[0].DONE.15);
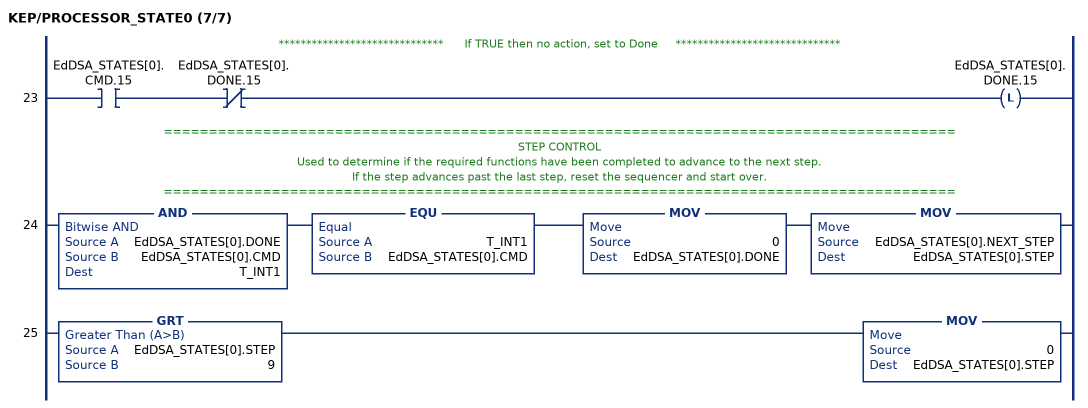
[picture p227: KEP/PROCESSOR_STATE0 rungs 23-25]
   // ******************************      If TRUE then no action, set to Done     ******************************
   23: XIC(EdDSA_STATES[0].CMD.15)XIO(EdDSA_STATES[0].DONE.15)OTL(EdDSA_STATES[0].DONE.15);
   // ========================================================================================
   // STEP CONTROL
   // Used to determine if the required functions have been completed to advance to the next step.
   // If the step advances past the last step, reset the sequencer and start over.
   // ========================================================================================
   24: AND(EdDSA_STATES[0].DONE,EdDSA_STATES[0].CMD,T_INT1)EQU(T_INT1,EdDSA_STATES[0].CMD)MOV(0,EdDSA_STATES[0].DONE)MOV(EdDSA_STATES[0].NEXT_STEP,EdDSA_STATES[0].STEP);
   25: GRT(EdDSA_STATES[0].STEP,9)MOV(0,EdDSA_STATES[0].STEP);
END_ROUTINE
